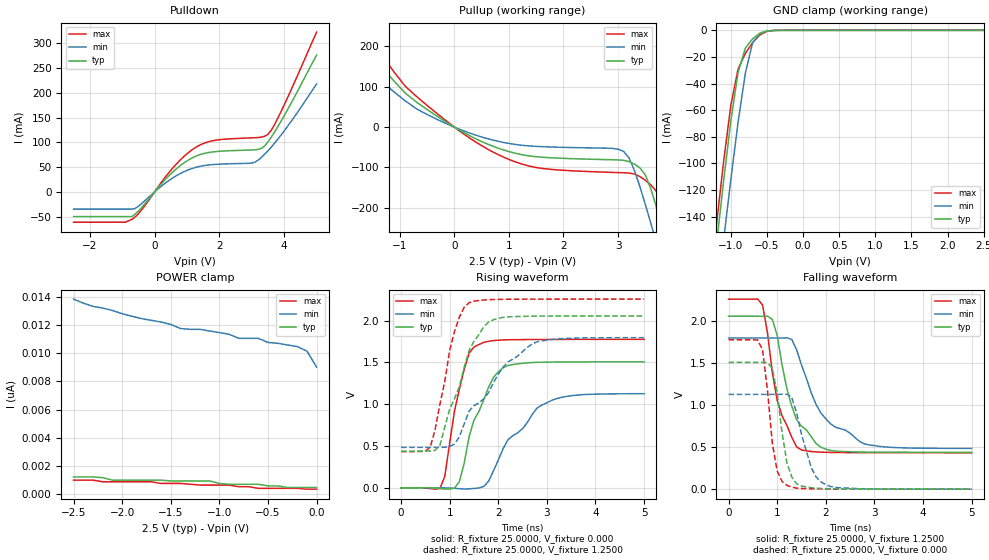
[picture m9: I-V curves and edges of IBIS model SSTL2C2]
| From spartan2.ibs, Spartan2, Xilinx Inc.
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|   Model SSTL2C2
[Model]   SSTL2C2
Model_type   I/O
Polarity   Non-Inverting
Enable   Active-Low
Vinl =   1.070V
Vinh =   1.430V
Vmeas =   1.2500V
Cref =  30.0000pF
| The Rref below represents only the parallel load, there is actually a series
| R, see the application notes for details.
Rref =  25.0000
Vref =   1.2500V
C_comp   6.5000pF   5.0000pF   8.0000pF
[Temperature Range]   27.0000   100.0000   0.000
[Voltage Range]   2.5000V   2.3750V   2.6250V
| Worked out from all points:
|   slope of the pulldown table from 0 to 0.375 V, typ, clamps not added: 13.3 ohm
|   slope of the pullup table from 0 to 0.375 V, typ, clamps not added: 13.5 ohm
|   GND clamp passes 1 mA (typ) near -0.53 V on its own axis
|   rising waveform, R_fixture 25.0000, V_fixture 0.000: 20-80 % time 501ps typ, 810ps min, 346ps max; typ from 0 V to 1.51 V
|   rising waveform, R_fixture 25.0000, V_fixture 1.2500: 20-80 % time 565ps typ, 996ps min, 379ps max; typ from 0.438 V to 2.06 V
|   falling waveform, R_fixture 25.0000, V_fixture 1.2500: 20-80 % time 455ps typ, 705ps min, 375ps max; typ from 2.06 V to 0.439 V
|   falling waveform, R_fixture 25.0000, V_fixture 0.000: 20-80 % time 229ps typ, 327ps min, 209ps max; typ from 1.51 V to 0 V
[Pulldown]
| voltage   I(typ)   I(min)   I(max)
-2.5V     -49.69mA   -34.66mA   -60.95mA
-900mV    -49.69mA   -34.66mA   -60.95mA
-700mV    -49.69mA   -34.66mA   -55.3mA
-400mV    -31.43mA   -23.28mA   -36.19mA
500mV     36.44mA    25.74mA    43.59mA
1.3V      72.85mA    50.1mA     91.09mA
1.9V      81.55mA    55.72mA    104.5mA
3V        84.69mA    58.35mA    109.1mA
3.3V      87.96mA    69.77mA    110.6mA
3.5V      100.9mA    82.99mA    116.3mA
4V        153.7mA    123.1mA    175.4mA
5V        276.1mA    217.6mA    322.4mA
[Pullup]
| voltage   I(typ)   I(min)   I(max)
-2.5V     327.4mA    250.2mA    392.3mA
-1.7V     206mA      155.7mA    248.4mA
-900mV    84.49mA    65.22mA    101.4mA
800mV     -52.07mA   -35.08mA   -67.97mA
3V        -81.26mA   -54.59mA   -112.7mA
3.2V      -85.38mA   -76.17mA   -113.8mA
3.4V      -100.9mA   -147.5mA   -122.5mA
3.6V      -152.8mA   -238.4mA   -143mA
3.7V      -196.7mA   -286.3mA   -159mA
3.8V      -244.6mA   -335.1mA   -190.1mA
4V        -346mA     -434.4mA   -281.1mA
5V        -880.7mA   -943.9mA   -818.2mA
[GND_clamp]
| voltage   I(typ)   I(min)   I(max)
-2.5V     -851.8mA   -860.9mA   -847.5mA
-1.2V     -161.8mA   -205.3mA   -146.7mA
-1.1V     -113.2mA   -157.8mA   -98.56mA
-1V       -68.04mA   -112mA     -56.27mA
-900mV    -31.6mA    -69.09mA   -29.2mA
-800mV    -13.5mA    -32.34mA   -17.42mA
-700mV    -6.408mA   -9.455mA   -9.303mA
-600mV    -2.237mA   -2.349mA   -3.538mA
-500mV    -423.5uA   -545.3uA   -698.2uA
-400mV    -42.44uA   -91.28uA   -59.93uA
2.5V      465.7pA    32.48nA    320.1pA
[POWER_clamp]
| voltage   I(typ)   I(min)   I(max)
-2.5V     1.222nA    13.85nA    989.5pA
-2.3V     1.222nA    13.33nA    989.5pA
-2.1V     989.5pA    13.04nA    873.1pA
-1.4V     931.3pA    11.76nA    756.7pA
-1.2V     931.3pA    11.7nA     640.3pA
-900mV    698.5pA    11.35nA    640.3pA
-800mV    698.5pA    11.06nA    523.9pA
-600mV    698.5pA    11.06nA    407.5pA
-500mV    582.1pA    10.77nA    407.5pA
-200mV    465.7pA    10.48nA    407.5pA
-100mV    465.7pA    10.16nA    349.2pA
0V        465.7pA    9.022nA    349.2pA
[Ramp]
| variable   typ   min   max
dV/dt_r   0.9042/0.5002n   0.6756/0.8377n   1.0656/0.3423n
dV/dt_f   0.9190/0.7247n   0.7164/1.1416n   1.0479/0.5134n
R_load = 25.0000
[Rising Waveform]
R_fixture = 25.0000
V_fixture = 0.000
| time   V(typ)   V(min)   V(max)
0s        2.219uV    0V         0V
800ps     -7.399mV   1.028mV    -7.234mV
900ps     -14.9mV    -547uV     138.2mV
1.2ns     74.01mV    -10.37mV   1.181V
1.5ns     811.1mV    -7.305mV   1.684V
1.8ns     1.204V     77.93mV    1.753V
2ns       1.388V     332.7mV    1.766V
2.2ns     1.464V     576.4mV    1.771V
2.9ns     1.502V     991.3mV    1.775V
5ns       1.507V     1.126V     1.776V
[Rising Waveform]
R_fixture = 25.0000
V_fixture = 1.2500
V_fixture_min = 1.1100
V_fixture_max = 1.3900
| time   V(typ)   V(min)   V(max)
0s        438.3mV    484.1mV    432.9mV
600ps     440.1mV    484.6mV    485.5mV
800ps     509.7mV    484.8mV    1V
1ns       941.2mV    495.1mV    1.644V
1.1ns     1.065V     524.6mV    1.871V
1.4ns     1.643V     917.7mV    2.214V
1.8ns     1.982V     1.138V     2.251V
2.2ns     2.045V     1.507V     2.256V
2.8ns     2.054V     1.748V     2.257V
5ns       2.056V     1.796V     2.258V
[Falling Waveform]
R_fixture = 25.0000
V_fixture = 1.2500
V_fixture_min = 1.1100
V_fixture_max = 1.3900
| time   V(typ)   V(min)   V(max)
0s        2.056V     1.797V     2.258V
700ps     2.055V     1.797V     2.188V
800ps     2.058V     1.797V     1.863V
900ps     2.019V     1.797V     1.387V
1ns       1.831V     1.796V     1.058V
1.2ns     1.196V     1.8V       758.4mV
1.4ns     826.9mV    1.658V     502.5mV
1.9ns     498.9mV    906.1mV    440.2mV
2.7ns     442mV      566.6mV    434.4mV
5ns       438.7mV    484.8mV    433.2mV
[Falling Waveform]
R_fixture = 25.0000
V_fixture = 0.000
| time   V(typ)   V(min)   V(max)
0s        1.507V     1.127V     1.776V
600ps     1.507V     1.127V     1.773V
700ps     1.508V     1.127V     1.657V
900ps     1.435V     1.127V     548.7mV
1ns       1.145V     1.127V     216.6mV
1.2ns     315.5mV    1.129V     46.19mV
1.3ns     145.2mV    1.091V     24.41mV
1.7ns     18.01mV    258.4mV    5.774mV
2ns       6.311mV    53.19mV    3.161mV
5ns       294.6uV    356.6uV    279.6uV
